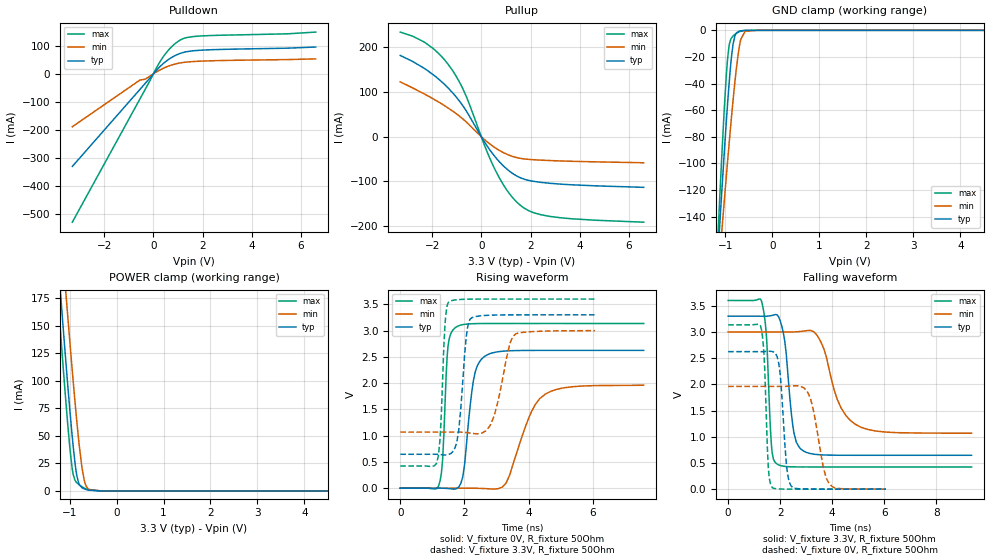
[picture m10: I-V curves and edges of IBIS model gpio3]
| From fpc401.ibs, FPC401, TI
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|   gpio3 Model
[Model]   gpio3
Model_type   I/O
Polarity   Non-Inverting
Enable   Active-Low
Vinl = 0.8
Vinh = 2
Vmeas = 1.65
Vref = 3.3
Cref = 2pF
Rref = 50
|   typ   min   max
|   (nom PVT)   (fast PVT)   (slow PVT)
C_comp   1.508e-12   1.472e-12   1.546e-12
| Where nom  PVT is Nominal Process, 3.3V, 27C
|   Fast PVT is Strong Process,  3.6V, -40C
|   Slow PVT is Weak Process,   3V, 125C
[Voltage Range]   3.3   3   3.6
|Junction Temperature
[Temperature Range]   27   125   -40
[Pullup Reference]   3.3   3   3.6
[Pulldown Reference]   0   0   0
[Power Clamp Reference]   3.3   3   3.6
[GND Clamp Reference]   0   0   0
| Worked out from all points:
|   slope of the pulldown table from 0 to 0.495 V, typ, clamps not added: 11.5 ohm
|   slope of the pullup table from 0 to 0.495 V, typ, clamps not added: 12.3 ohm
|   GND clamp passes 1 mA (typ) near -0.73 V on its own axis
|   POWER clamp passes 1 mA (typ) near -0.62 V on its own axis
|   falling waveform, V_fixture 3.3V, R_fixture 50Ohm: 20-80 % time 307ps typ, 745ps min, 171ps max; typ from 3.3 V to 0.646 V
|   rising waveform, V_fixture 0V, R_fixture 50Ohm: 20-80 % time 280ps typ, 703ps min, 135ps max; typ from 0 V to 2.62 V
|   rising waveform, V_fixture 3.3V, R_fixture 50Ohm: 20-80 % time 206ps typ, 402ps min, 129ps max; typ from 0.646 V to 3.3 V
|   falling waveform, V_fixture 0V, R_fixture 50Ohm: 20-80 % time 215ps typ, 427ps min, 137ps max; typ from 2.62 V to 0 V
[Pulldown]
|   Voltage   I(typ)   I(min)   I(max)
-3.3V     -329.6mA   -188.3mA   -528.3mA
-552mV    -55.54mA   -22.16mA   -89.62mA
-330mV    -33.39mA   -18.81mA   -54.18mA
153mV     15.81mA    8.562mA    26.43mA
381mV     35.36mA    19.17mA    58.75mA
580.8mV   49.31mA    26.71mA    81.67mA
922.8mV   66.96mA    36.02mA    110.7mA
1.251V    77.19mA    41.11mA    126.9mA
1.722V    83.06mA    44.51mA    133.8mA
5.441V    91.55mA    50.91mA    142.7mA
6.6V      95.65mA    53.4mA     148.8mA
[GND Clamp]
|   Voltage   I(typ)   I(min)   I(max)
-3.3V     -1.513A    -1.193A    -1.906A
-1.197V   -191.2mA   -204.5mA   -183.5mA
-1.115V   -143.1mA   -168mA     -122mA
-1.076V   -120.9mA   -150.9mA   -94.02mA
-985.2mV  -71.44mA   -112mA     -36.5mA
-924mV    -41.43mA   -86.62mA   -12.38mA
-838.2mV  -10.76mA   -53.2mA    -4.293mA
-720mV    -792.9uA   -16.02mA   -1.349mA
-672mV    -334.3uA   -6.9mA     -676.3uA
-582mV    -58.47uA   -755.9uA   -116.5uA
-330mV    -100.8nA   -785.8nA   -64.34nA
6.6V      0A         0A         0A
[Pullup]
|   Voltage   I(typ)   I(min)   I(max)
-3.3V     182mA      122.9mA    234.3mA
-2.244V   150.2mA    93.51mA    209mA
-1.734V   128.8mA    77.57mA    186.2mA
-1.211V   100.9mA    59mA       151.4mA
-620.4mV  58.34mA    33.49mA    91.03mA
165mV     -14.93mA   -8.222mA   -24.57mA
660mV     -51.63mA   -28.25mA   -84.9mA
1.15V     -77.44mA   -41.75mA   -128.1mA
1.647V    -93.19mA   -48.99mA   -156.2mA
2.143V    -100mA     -51.54mA   -170.4mA
2.832V    -104.4mA   -53.42mA   -178.7mA
6.6V      -113.3mA   -58.24mA   -191.3mA
[POWER Clamp]
|   Voltage   I(typ)   I(min)   I(max)
-3.3V     1.467A     1.487A     1.482A
-1.284V   231.6mA    292.9mA    198mA
-1.154V   158.7mA    221.3mA    123mA
-1.092V   124.6mA    187.5mA    88.46mA
-1.036V   94.8mA     157.5mA    59.05mA
-992.4mV  72.91mA    135mA      38.7mA
-920.4mV  39.63mA    98.64mA    14.6mA
-805.2mV  6.967mA    46.05mA    5.92mA
-687mV    1.903mA    9.647mA    2.597mA
-591mV    686.4uA    1.392mA    876.3uA
-330mV    2.458uA    8.051uA    1.192uA
6.6V      0A         0A         0A
[Ramp]
R_load = 50
|   typ   min   max
dV/dt_r   1.57408/2.80331e-10   1.17609/7.03084e-10   1.88135/1.34991e-10
dV/dt_f   1.59248/3.07357e-10   1.15907/7.4466e-10   1.90604/1.71452e-10
[Falling Waveform]
V_fixture = 3.3V
V_fixture_min = 3V
V_fixture_max = 3.6V
R_fixture = 50Ohm
|   Time   V(typ)   V(min)   V(max)
0s        3.3V       3V         3.6V
1.284ns   3.299V     3V         3.586V
1.485ns   3.3V       3V         2.822V
1.662ns   3.311V     3V         858.5mV
1.869ns   3.326V     3V         483.9mV
2.54ns    1.05V      3V         424.8mV
2.806ns   760.6mV    3.01V      423.3mV
3.505ns   656.9mV    2.867V     423.1mV
4.887ns   646.3mV    1.239V     423.2mV
9.364ns   646.4mV    1.068V     423mV
[Rising Waveform]
V_fixture = 0V
V_fixture_min = 0V
V_fixture_max = 0V
R_fixture = 50Ohm
|   Time   V(typ)   V(min)   V(max)
0s        471.7pV    23.62nV    109.5pV
1.188ns   1.001mV    81.35nV    35.03mV
1.319ns   704.7uV    2.255uV    532.7mV
1.485ns   -5.762mV   -8.709uV   2.68V
1.74ns    -9.814mV   15.09uV    3.066V
2.283ns   2.059V     472.7uV    3.132V
2.625ns   2.507V     -6.485mV   3.135V
3.299ns   2.613V     97.41mV    3.135V
4.523ns   2.623V     1.793V     3.136V
7.587ns   2.623V     1.96V      3.135V
[Rising Waveform]
V_fixture = 3.3V
V_fixture_min = 3V
V_fixture_max = 3.6V
R_fixture = 50Ohm
|   Time   V(typ)   V(min)   V(max)
0s        646.2mV    1.068V     423.1mV
1.129ns   646mV      1.068V     470.5mV
1.242ns   641.5mV    1.068V     942.1mV
1.407ns   632.8mV    1.068V     3.207V
1.514ns   642.2mV    1.068V     3.545V
1.824ns   1.108V     1.069V     3.59V
2.181ns   3.22V      1.05V      3.599V
2.798ns   3.293V     1.188V     3.6V
3.594ns   3.3V       2.937V     3.6V
6.072ns   3.3V       3V         3.6V
[Falling Waveform]
V_fixture = 0V
V_fixture_min = 0V
V_fixture_max = 0V
R_fixture = 50Ohm
|   Time   V(typ)   V(min)   V(max)
0s        2.623V     1.96V      3.136V
1.242ns   2.623V     1.96V      3.119V
1.384ns   2.625V     1.96V      2.527V
1.541ns   2.63V      1.96V      442.6mV
1.694ns   2.625V     1.96V      31.2mV
1.947ns   2.401V     1.96V      4.249mV
2.431ns   55.49mV    1.968V     594uV
3.176ns   960.2uV    1.716V     -22.44uV
3.879ns   -10.85uV   110.1mV    37.39uV
6.072ns   190.7uV    180.4uV    8.466uV
